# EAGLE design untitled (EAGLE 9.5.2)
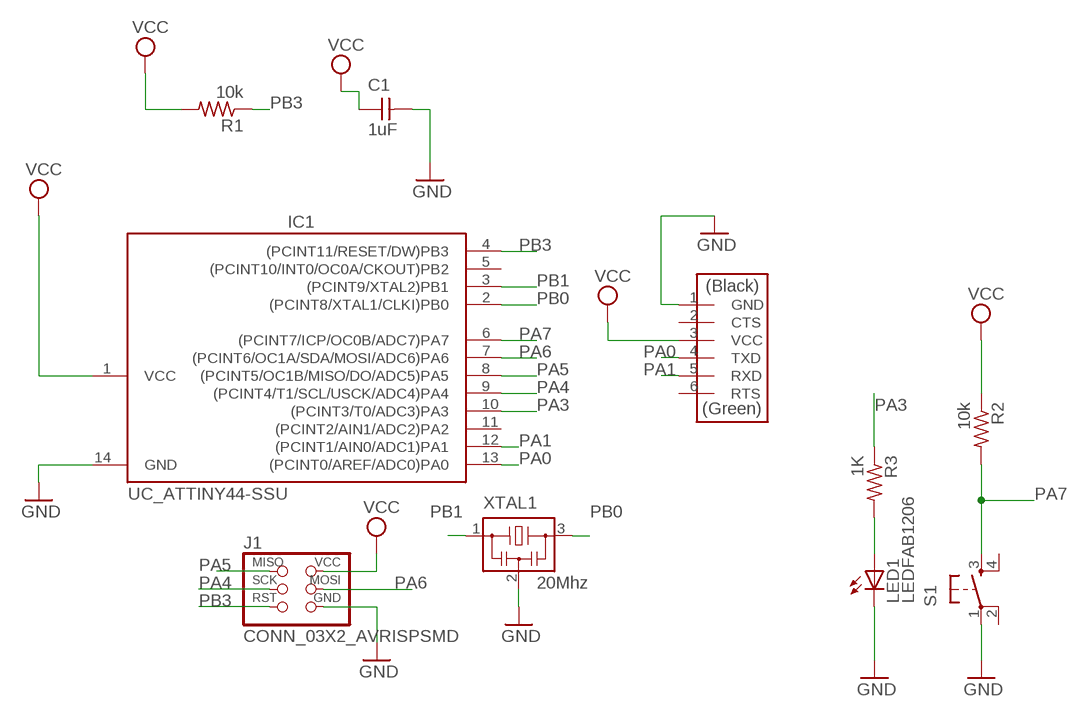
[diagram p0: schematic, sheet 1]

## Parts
C1  1uF  CAP_UNPOLARIZEDFAB  [C1206FAB]
IC1  UC_ATTINY44-SSU  [SOIC14]
J1  CONN_03X2_AVRISPSMD  [2X03SMD]
J2  CONN_06_FTDI-SMD-HEADER  [1X06SMD]
LED1  LEDFAB1206  [LED1206FAB]
R1  10k  R1206FAB  [R1206FAB]
R2  10k  R1206FAB  [R1206FAB]
R3  1K  R1206FAB  [R1206FAB]
S1  SW_SWITCH_TACTILE_6MM6MM_SWITCH  [6MM_SWITCH]
XTAL1  20Mhz  XTAL_RESONATOR  [EFOBM]

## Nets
GND: C1.2 IC1.14(GND) J1.6(GND) J2.1(GND) LED1.2(C) S1.1(P) XTAL1.2
N$1: LED1.1(A) R3.2
PA0: IC1.13((PCINT0/AREF/ADC0)PA0) J2.4(TXD)
PA1: IC1.12((PCINT1/AIN0/ADC1)PA1) J2.5(RXD)
PA3: IC1.10((PCINT3/T0/ADC3)PA3) R3.1
PA4: IC1.9((PCINT4/T1/SCL/USCK/ADC4)PA4) J1.3(SCK)
PA5: IC1.8((PCINT5/OC1B/MISO/DO/ADC5)PA5) J1.1(MISO)
PA6: IC1.7((PCINT6/OC1A/SDA/MOSI/ADC6)PA6) J1.4(MOSI)
PA7: IC1.6((PCINT7/ICP/OC0B/ADC7)PA7) R2.2 S1.3(S)
PB0: IC1.2((PCINT8/XTAL1/CLKI)PB0) XTAL1.3
PB1: IC1.3((PCINT9/XTAL2)PB1) XTAL1.1
PB3: IC1.4((PCINT11/RESET/DW)PB3) J1.5(RST) R1.1
VCC: C1.1 IC1.1(VCC) J1.2(VCC) J2.3(VCC) R1.2 R2.1
Unconnected: IC1.5((PCINT10/INT0/OC0A/CKOUT)PB2) IC1.11((PCINT2/AIN1/ADC2)PA2) J2.2(CTS) J2.6(RTS) S1.2(P1) S1.4(S1)

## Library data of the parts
C1 = fab:CAP_UNPOLARIZED
IC1 = fab:UC_ATTINY44
J1 = fab:CONN_03X2_AVRISP
J2 = fab:CONN_06_FTDI-SMD-HEADER
LED1 = fab:LED: LED
R1-R3 = fab:R: Resistor (US Symbol)
S1 = fab:SW_SWITCH_TACTILE_6MM: OMRON SWITCH
XTAL1 = fab:XTAL_RESONATOR

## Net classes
0 default: width 0.406 mm

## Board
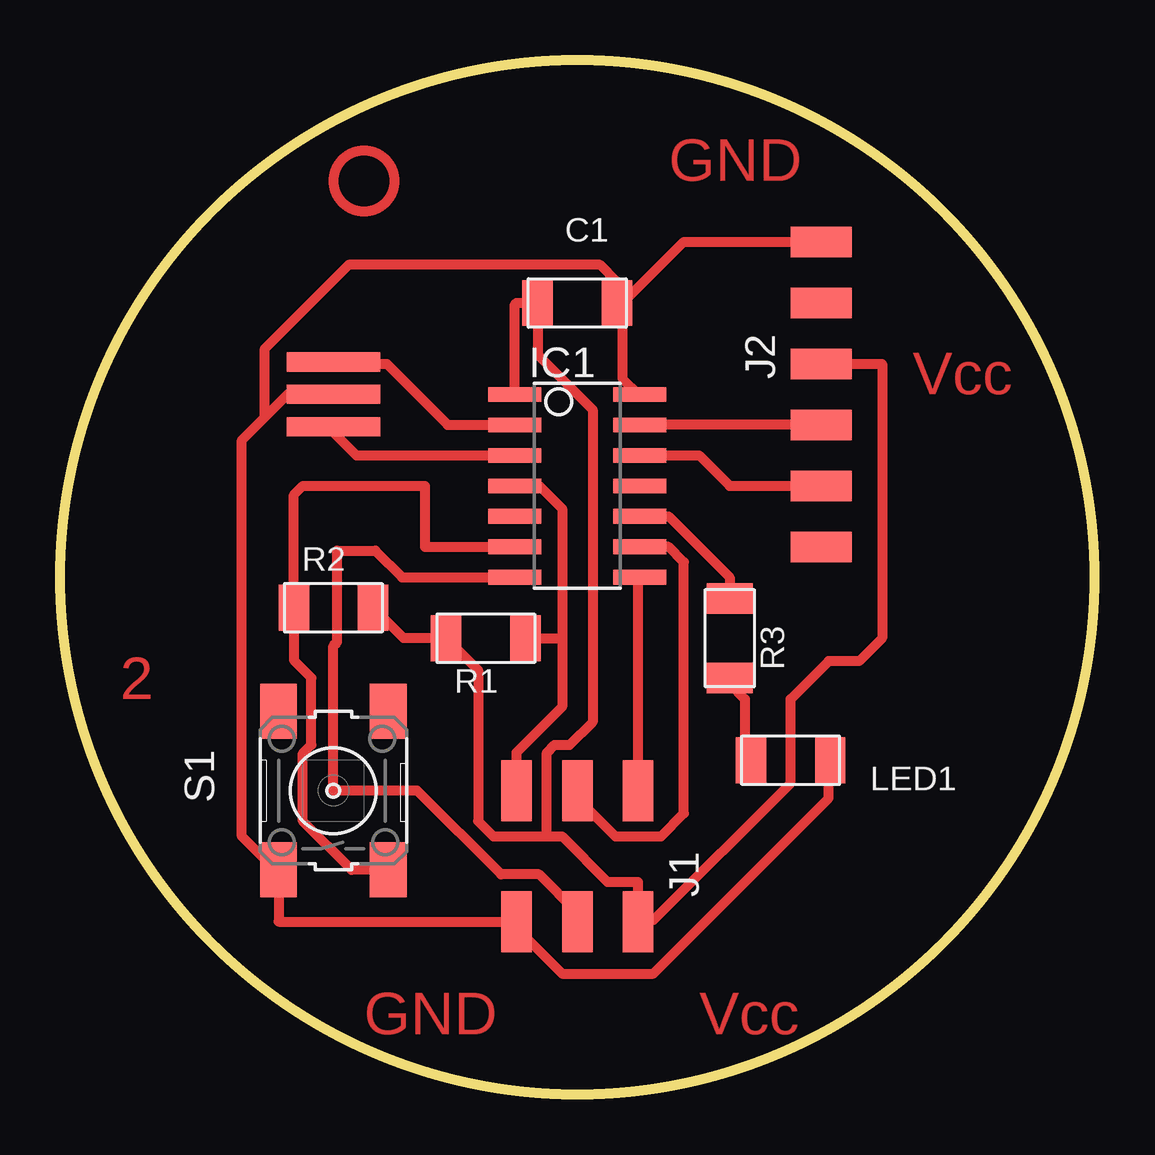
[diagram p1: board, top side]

Size 43.11 x 43.11 mm. Coordinates in mm from the lower left corner, seen from the top.
Outline: circle at 21.55,21.55 radius 21.55
Copper layers (1*16): Top 0.035mm / dielectric 1.5mm / Bottom 0.035mm
Design rules "fab *": minimum track width 10mil, minimum drill 32mil, track to track 0.4mm, track to pad 0.4mm, pad to pad 0.4mm, via to via 16mil, smd to smd 6mil, copper to edge 16mil, drill to drill 16mil, minimum pad ring 10mil, minimum via ring 8mil, stop-mask expansion 4mil, vias tented up to drill 0mil, thermal gap 16mil

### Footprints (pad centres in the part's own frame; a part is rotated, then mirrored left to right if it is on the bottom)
C1206FAB = smd 1.27 x 1.905: 1 -1.651,0; 2 1.651,0
SOIC14 = smd 0.61 x 2.21: 1 -3.81,-2.603; 2 -2.54,-2.603; 3 -1.27,-2.603; 4 0,-2.603; 5 1.27,-2.603; 6 2.54,-2.603; 7 3.81,-2.603; 8 3.81,2.603; 9 2.54,2.603; 10 1.27,2.603; 11 0,2.603; 12 -1.27,2.603; 13 -2.54,2.603; 14 -3.81,2.603
2X03SMD = smd 2.54 x 1.27: 1 -2.54,2.54; 2 2.92,2.54; 3 -2.54,0; 4 2.92,0; 5 -2.54,-2.54; 6 2.92,-2.54
1X06SMD = smd 2.54 x 1.27: 1 0,6.35; 2 0,3.81; 3 0,1.27; 4 0,-1.27; 5 0,-3.81; 6 0,-6.35
LED1206FAB = smd 1.27 x 1.905: 1 -1.651,0; 2 1.651,0
R1206FAB = smd 1.27 x 1.905: 1 -1.651,0; 2 1.651,0
6MM_SWITCH = smd 2.286 x 1.524: 1 -3.302,2.286; 2 3.302,2.286; 3 -3.302,-2.286; 4 3.302,-2.286
EFOBM = smd 0.8 x 3.9: 1 -1.35,0; 2 0,0; 3 1.35,0

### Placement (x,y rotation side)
C1  21.55,32.98 0 top
IC1  21.55,25.36 270 top
J1  21.55,10.12 270 top
J2  31.71,29.17 0 top
LED1  30.44,13.93 0 top
R1  17.74,19.01 180 top
R2  11.39,20.28 180 top
R3  27.9,19.01 270 top
S1  11.39,12.66 90 top
XTAL1  11.39,29.17 90 top

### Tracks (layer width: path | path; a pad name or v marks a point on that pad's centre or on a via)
GND
  Top 0.406: 23.46,32.98 23.46,29.81 24.09,29.17 IC1.14 | J2.1 26,35.52 23.46,32.98 | 23.46,32.98 C1.2 23.2,33.87 22.5,34.57 12.03,34.57 8.54,31.08 8.54,28.22 | LED1.2 32.03,13.93 32.03,12.34 24.73,5.04 20.92,5.04 19.01,6.95 J1.6 9.11,7.2 S1.1 8.85,9.49 7.58,10.76 7.58,27.27 8.54,28.22 | XTAL1.2 9.49,29.17 8.54,28.22
N$1
  Top 0.406: LED1.1 28.54,13.93 28.54,16.47 27.9,17.11 R3.2
PA0
  Top 0.406: J2.4 IC1.13
PA1
  Top 0.406: IC1.12 26.63,26.63 27.9,25.36 J2.5
PA3
  Top 0.406: R3.1 27.9,21.55 25.36,24.09 IC1.10
PA4
  Top 0.406: IC1.9 25.36,22.82 26,22.19 26,11.71 25.05,10.76 23.14,10.76 21.55,12.34 J1.3
PA5
  Top 0.406: J1.1 24.09,21.55 IC1.8
PA6
  Top 0.406: IC1.7 14.25,21.55 13.14,22.66 11.55,22.66 11.55,18.85 11.39,18.69 11.39,12.66 14.88,12.66 18.38,9.17 19.97,9.17 21.55,7.58 J1.4
PA7
  Top 0.406: S1.3 12.15,9.36 10.12,11.39 10.12,14.21 10.48,14.57 10.48,17.36 9.74,18.1 R2.2 9.74,24.98 10.12,25.36 15.2,25.36 15.2,22.82 IC1.6
PB0
  Top 0.406: IC1.2 16.15,27.9 13.61,30.44 11.39,30.44 XTAL1.3
PB1
  Top 0.406: IC1.3 12.34,26.63 11.39,27.59 XTAL1.1
PB3
  Top 0.406: J1.5 19.01,14.25 20.92,16.16 20.92,19.01 | IC1.4 19.97,25.36 20.92,24.41 20.92,19.01 | R1.1 20.92,19.01
VCC
  Top 0.406: 20.28,10.76 18.06,10.76 17.42,11.39 17.42,17.68 R1.2 14.31,19.01 R2.1 | 20.28,10.76 20.92,10.76 22.82,8.85 24.09,8.85 J1.2 24.09,7.27 24.73,7.27 30.44,12.98 30.44,16.47 32.03,18.06 33.3,18.06 34.25,19.01 34.25,30.44 J2.3 | 20.28,10.76 20.28,14.25 20.6,14.57 21.24,14.57 22.19,15.52 22.19,28.54 19.9,30.82 C1.1 19.01,32.98 18.95,32.92 IC1.1
(copper drawn outside any net)
  shapes: Top circle x1

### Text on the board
Top: GND | Vcc | 2 | GND | Vcc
